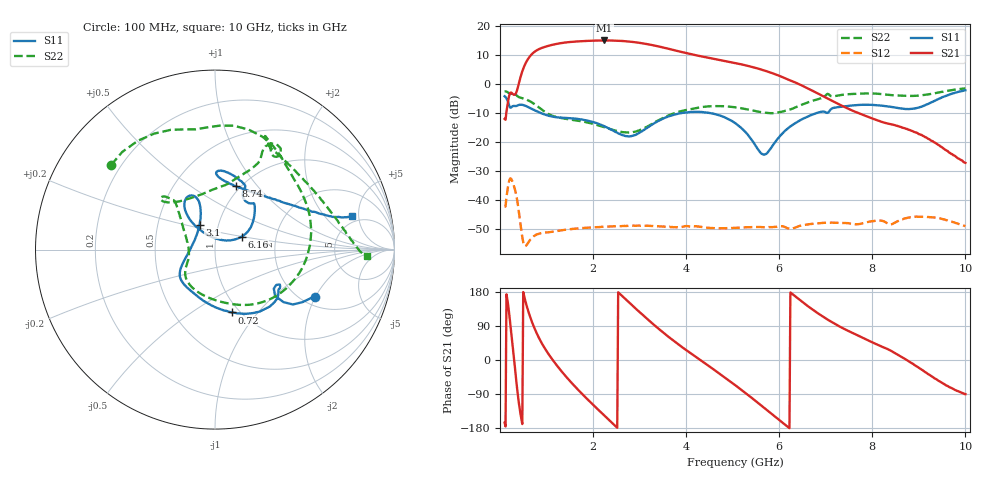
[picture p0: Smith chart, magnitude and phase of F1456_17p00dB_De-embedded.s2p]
! Integrated Device Technology
! Corporate Headquarters
! 6024 Silver Creek Valley Road
! San Jose, CA 95138  USA
! Phone:  1-408-284-8200
! Toll Free:  1-800-223-1366
! Webpage:  http://www.idt.com/
! Timing and RF Division
! 515 Groton Road, Suite 102
! Westford, MA 01886-6024
! Device:  F1456
! Description: 6-bit 0.5 dB Transmit Variable Gain Amplifier
! Frequency:  2100.0 -  2950.00 MHz
! Package:  6x6 mm Thin QFN Plastic Package: 28 pin
! State:  34
! Atten State:  17.0 dB
! Voltage:  +5.00 Volts
! Current:  216.996 mA
! Data:  The device was measured on a the F1455 evaluation board which has
!  individual transmission lines to the RF pins.  Data was collected
!  using a calibrated network analyzer.  The evaluation board was
!  de-embedded using a TRL calibration technique.
!  The reference plane is the edge of the package pin.
!  Pin  1 = CSb
!  Pin  2 = DATA
!  Pin  3 = CLK
!  Pin  4 = RSET
!  Pin  5 = GND
!  Pin  6 = RFIN  = Port 1
!  Pin  7 = GND
!  Pin  8 = NC
!  Pin  9 = NC
!  Pin 10 = NC
!  Pin 11 = NC
!  Pin 12 = NC
!  Pin 13 = NC
!  Pin 14 = /STBY
!  Pin 15 = GND
!  Pin 16 = RFOUT  = Port 2
!  Pin 17 = GND
!  Pin 18 = NC
!  Pin 19 = NC
!  Pin 20 = NC
!  Pin 21 = GND
!  Pin 22 = NC
!  Pin 23 = GND
!  Pin 24 = NC
!  Pin 25 = NC
!  Pin 26 = NC
!  Pin 27 = GND
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# GHz S dB R 50
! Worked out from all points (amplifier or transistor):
!   496 points, 100 MHz to 10 GHz, reference 50 ohm
!   highest |S21| = 15.1 dB at 2.24 GHz (marker M1)
!   |S21| within 3 dB of that: 837.3 MHz to 3.652 GHz (2.815 GHz wide, 125 % of centre)
!   unconditionally stable (mu >= 1): start of sweep to end of sweep
!   at 1.74 GHz: K = 24.98, MAG = 15.4 dB, |S12| = -49.8 dB
!   at 5.06 GHz: K = 53.24, MAG = 8.2 dB, |S12| = -49.7 dB
!   at 10 GHz: K = 359.07, MAG = -17.6 dB, |S12| = -49.1 dB
!   S11 on the Smith chart (normalised r, x): 100 MHz: 2.36, -1.99; 720 MHz: 0.92, -0.74; 3.1 GHz: 0.81, +0.23; 6.16 GHz: 1.33, +0.20; 8.74 GHz: 0.95, +0.78; 10 GHz: 4.21, +4.08
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0.1  -4.19 -25.1  -12.03 -165.5  -42.29 48.6  -2.54 140.8
0.32  -7.56 -31.4  -3.64 -17.9  -36.36 -149.3  -3.32 67.1
0.44  -7.09 -41.2  2.36 -141.7  -48.31 135.8  -4.67 37.9
0.56  -7.57 -56.8  7.52 149.1  -55.89 157.9  -5.25 10.9
0.72  -8.82 -75.1  10.90 90.3  -52.73 140.7  -6.67 -24.0
0.96  -10.48 -99.1  12.87 31.5  -51.35 96.1  -9.53 -67.2
1.18  -11.37 -116.2  13.81 -7.6  -50.95 71.6  -11.21 -93.9
1.48  -11.75 -132.6  14.55 -52.3  -50.21 47.3  -12.14 -119.8
1.76  -12.23 -143.3  14.88 -88.9  -49.77 29.6  -12.84 -134.9
2.24  -14.53 -159.0  15.12 -146.3  -49.33 4.6  -14.86 -151.2
2.64  -17.68 172.0  14.93 167.2  -49.06 -14.6  -16.60 -168.9
3.1  -15.77 121.9  14.03 115.2  -48.94 -36.7  -15.22 157.4
3.4  -12.73 110.3  13.08 83.3  -49.12 -51.0  -12.58 141.3
3.74  -10.58 109.0  11.77 49.8  -49.46 -65.1  -10.05 131.9
4.1  -9.62 114.0  10.37 17.7  -49.32 -81.1  -8.60 130.7
5.06  -13.53 130.1  7.30 -66.9  -49.73 -125.1  -8.02 137.2
5.66  -24.34 77.9  4.84 -124.7  -49.47 -159.5  -9.81 120.6
6.16  -15.63 26.1  1.81 -174.4  -49.72 168.4  -9.07 84.8
6.7  -10.62 41.7  -2.16 134.5  -48.34 143.4  -5.84 64.8
8.36  -7.75 87.9  -13.71 26.9  -48.49 71.6  -3.73 62.4
8.74  -8.58 71.7  -15.46 -0.0  -46.30 64.9  -4.05 49.1
10  -2.11 13.7  -27.21 -90.1  -49.11 -22.3  -1.46 -2.6
